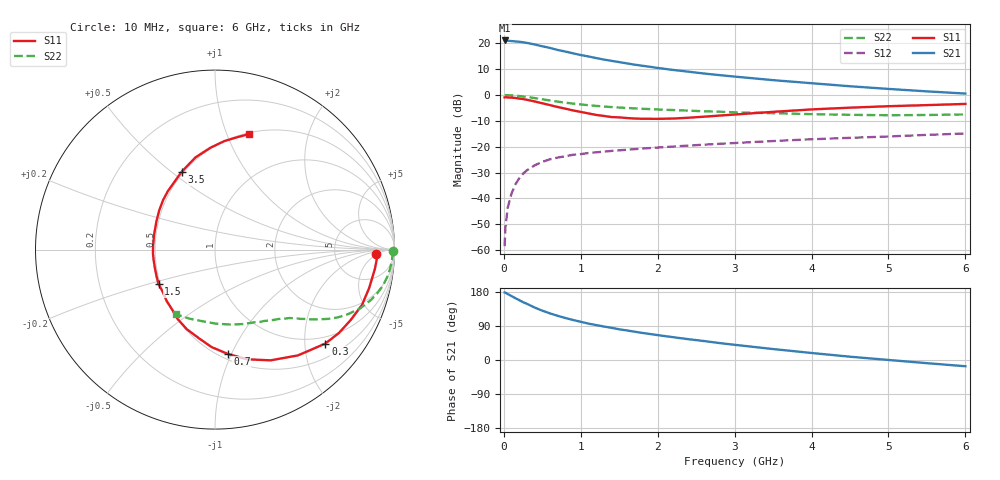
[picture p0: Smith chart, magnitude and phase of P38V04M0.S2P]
! SIEMENS Small Signal Semiconductors
! BFP181
! Si NPN RF Bipolar Junction Transistor in SOT143
! VCE = 8 V  IC = 4 mA
! Common Emitter S-Parameters:  March  1996
# GHz  S  MA  R  50
!  f  S11  S21  S12  S22
! GHz  MAG  ANG  MAG  ANG  MAG  ANG  MAG  ANG
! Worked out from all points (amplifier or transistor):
!   36 points, 10 MHz to 6 GHz, reference 50 ohm
!   highest |S21| = 21.1 dB at 10 MHz (marker M1)
!   |S21| within 3 dB of that: start of sweep to 614.9 MHz
!   unconditionally stable (mu >= 1): 2.014 GHz to end of sweep
!   at 250 MHz: K = 0.18, MSG = 25.4 dB, |S12| = -30.4 dB
!   at 1.4 GHz: K = 0.81, MSG = 17.4 dB, |S12| = -21.6 dB
!   at 6 GHz: K = 1.07, MAG = 6.0 dB, |S12| = -14.9 dB
!   S11 on the Smith chart (normalised r, x): 10 MHz: 17, -4; 300 MHz: 0.82, -2.48; 700 MHz: 0.55, -0.97; 1.5 GHz: 0.49, -0.22; 3.5 GHz: 0.49, +0.54; 6 GHz: 0.51, +1.20
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0.01  0.8973 -1.6  11.29 178.3  0.0012 86.0  0.991 -0.6
0.02  0.9043 -2.7  11.26 177.8  0.0027 85.2  0.9886 -1.2
0.05  0.8977 -6.7  11.13 174.2  0.0066 90.4  0.9884 -3.2
0.1  0.8854 -13.9  10.98 168.7  0.0125 80.4  0.9811 -6.4
0.2  0.8519 -27.4  10.67 157.9  0.0246 74.7  0.955 -12.4
0.25  0.832 -34.0  10.39 152.6  0.0302 70.7  0.9347 -15.2
0.3  0.8075 -40.4  10.13 148.2  0.035 67.7  0.9147 -17.7
0.4  0.7491 -51.9  9.438 138.5  0.0437 61.8  0.8712 -22.2
0.5  0.6906 -63.3  8.711 130.2  0.051 56.9  0.8247 -25.8
0.6  0.6369 -73.7  8.1 123.0  0.0571 52.8  0.7817 -28.9
0.7  0.5849 -83.1  7.391 116.6  0.0618 49.5  0.7425 -31.3
0.9  0.5019 -100.3  6.368 105.6  0.07 44.7  0.6809 -34.8
1.1  0.4397 -118.1  5.54 96.0  0.0756 41.3  0.6331 -37.6
1.3  0.3934 -133.1  4.829 88.4  0.0803 38.9  0.5984 -39.9
1.5  0.3689 -148.4  4.313 81.1  0.0851 37.1  0.5704 -42.0
1.8  0.3468 -170.6  3.666 71.5  0.092 35.7  0.5407 -45.3
2.2  0.35 165.3  3.041 60.2  0.1008 33.5  0.5109 -50.0
2.8  0.3993 136.5  2.419 44.8  0.1138 30.6  0.4747 -58.1
3.5  0.4719 113.2  1.932 28.9  0.1288 27.1  0.4439 -69.2
4.5  0.5679 92.6  1.472 8.7  0.1485 21.1  0.4131 -88.9
5.5  0.6362 79.2  1.173 -8.4  0.1694 16.2  0.41 -110.1
6  0.671 73.6  1.063 -16.5  0.1801 12.9  0.4204 -121.0
